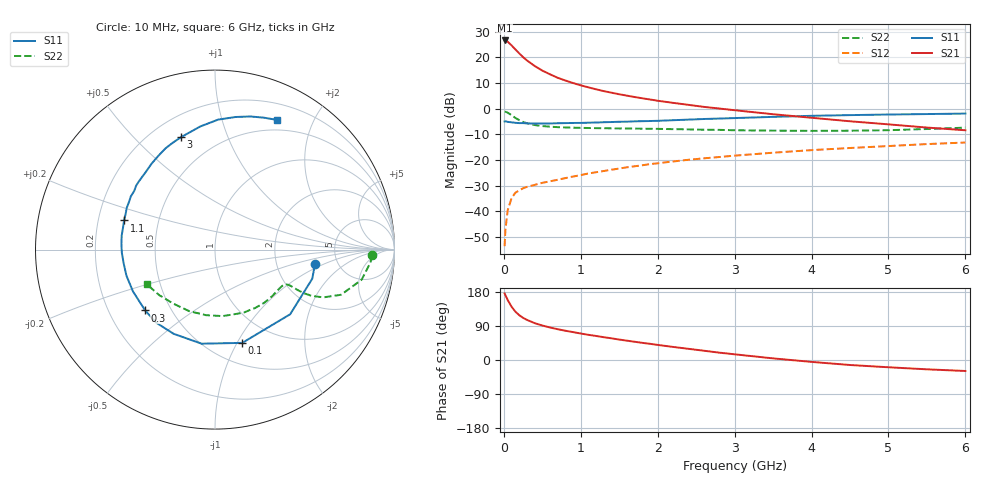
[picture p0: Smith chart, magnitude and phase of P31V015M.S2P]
! SIEMENS Small Signal Semiconductors
! BFP181
! Si NPN RF Bipolar Junction Transistor in SOT143
! VCE = 1 V  IC = 15 mA
! Common Emitter S-Parameters:  March  1996
# GHz  S  MA  R  50
!  f  S11  S21  S12  S22
! GHz  MAG  ANG  MAG  ANG  MAG  ANG  MAG  ANG
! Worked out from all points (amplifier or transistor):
!   36 points, 10 MHz to 6 GHz, reference 50 ohm
!   highest |S21| = 26.5 dB at 10 MHz (marker M1)
!   |S21| within 3 dB of that: start of sweep to 134.3 MHz
!   unconditionally stable (mu >= 1): start of sweep to 19.33 MHz; 311.3 MHz to end of sweep
!   at 250 MHz: K = 0.85, MSG = 25.5 dB, |S12| = -31.0 dB
!   at 1.4 GHz: K = 2.04, MAG = 9.2 dB, |S12| = -23.8 dB
!   at 6 GHz: K = 1.74, MAG = -2.6 dB, |S12| = -13.2 dB
!   S11 on the Smith chart (normalised r, x): 10 MHz: 3.36, -0.81; 100 MHz: 0.71, -1.05; 300 MHz: 0.36, -0.33; 1.1 GHz: 0.31, +0.14; 3 GHz: 0.32, +0.69; 6 GHz: 0.38, +1.52
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0.01  0.563 -8.4  21.24 175.6  0.0021 77.4  0.8753 -2.1
0.02  0.5656 -16.7  21.16 171.4  0.0043 76.2  0.869 -4.8
0.05  0.5524 -40.7  20.08 158.3  0.0105 74.4  0.8339 -11.6
0.1  0.5414 -73.7  17.05 140.8  0.018 57.5  0.7464 -19.7
0.15  0.5295 -98.1  14.2 127.6  0.0231 50.3  0.6597 -23.8
0.2  0.5227 -116.2  11.9 118.3  0.0256 47.6  0.5963 -25.6
0.25  0.5228 -128.9  10.06 111.2  0.0281 44.6  0.5513 -26.1
0.3  0.516 -138.9  8.693 105.9  0.0299 43.0  0.5191 -26.1
0.4  0.513 -152.9  6.776 97.3  0.0328 43.2  0.4792 -25.7
0.5  0.5144 -163.6  5.5 91.0  0.0359 43.7  0.4578 -25.6
0.6  0.5147 -171.6  4.66 85.8  0.0385 45.0  0.4451 -25.9
0.7  0.5195 -178.2  3.981 81.3  0.0412 46.5  0.4359 -26.4
0.8  0.5227 176.0  3.525 77.2  0.0444 47.6  0.4302 -27.3
1  0.527 166.4  2.838 69.9  0.0508 49.4  0.4222 -29.7
1.1  0.5321 162.2  2.594 66.4  0.0547 50.2  0.4195 -31.0
1.5  0.5548 147.8  1.904 53.9  0.0682 51.0  0.4118 -37.5
2.2  0.5949 126.5  1.295 34.5  0.0936 49.0  0.3982 -51.5
3  0.6547 106.7  0.931 15.0  0.1215 43.9  0.3792 -70.1
3.5  0.691 96.8  0.778 4.3  0.1387 40.3  0.3729 -83.5
4.5  0.7476 81.2  0.567 -13.2  0.1712 31.6  0.3717 -112.8
5.5  0.7838 69.7  0.428 -24.6  0.2041 23.1  0.4009 -140.7
6  0.8007 64.5  0.379 -29.0  0.2189 18.2  0.4262 -153.0
